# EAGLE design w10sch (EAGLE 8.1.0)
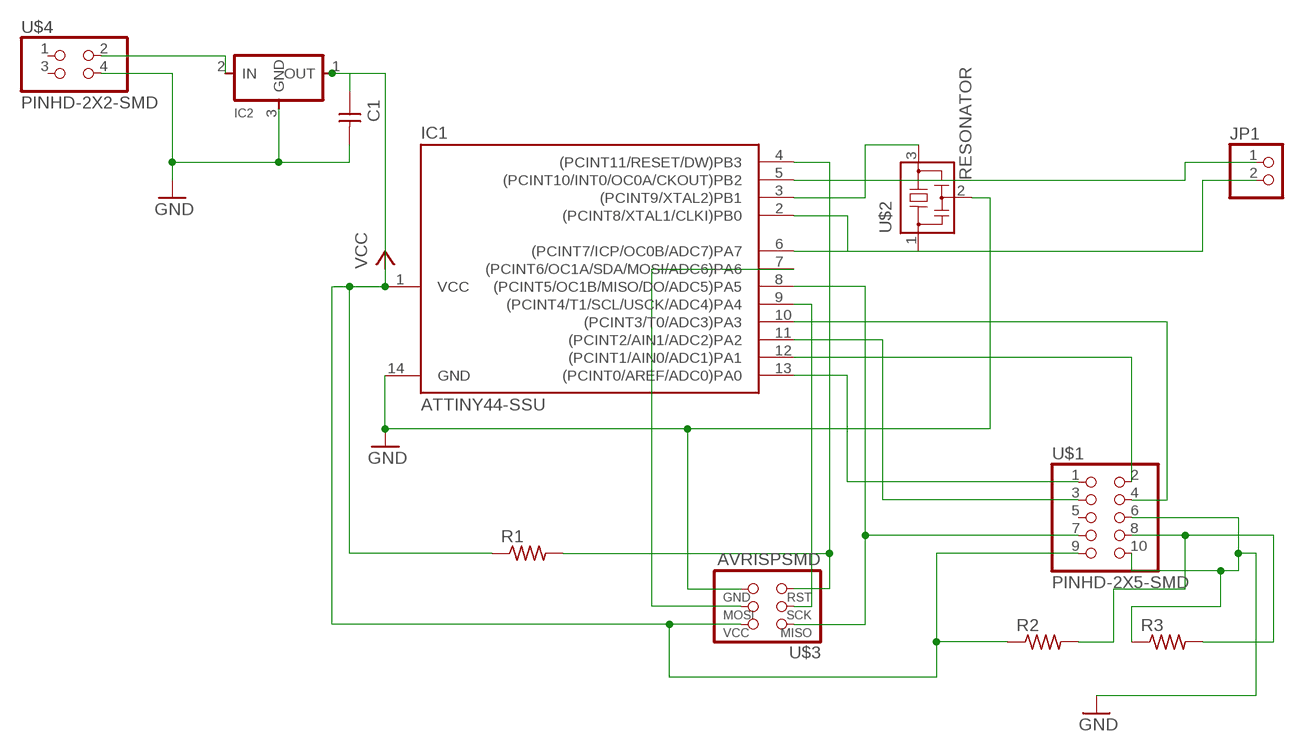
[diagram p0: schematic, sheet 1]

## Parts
C1  CAP-UNPOLARIZEDFAB  [C1206FAB]
IC1  ATTINY44-SSU  [SOIC14]
IC2  REGULATORSOT23  [SOT23]
JP1  PINHD-1X2  [1X02]
R1  RES-US1206FAB  [R1206FAB]
R2  RES-US1206FAB  [R1206FAB]
R3  RES-US1206FAB  [R1206FAB]
U$1  PINHD-2X5-SMD  [2X05SMD]
U$2  RESONATOR  [EFOBM]
U$3  AVRISPSMD  [2X03SMD]
U$4  PINHD-2X2-SMD  [2X02SMD]

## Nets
GND: C1.2 IC1.14(GND) IC2.3(GND) R3.1 U$1.6 U$1.10 U$2.2 U$3.6(GND) U$4.4
N$1: IC1.2((PCINT8/XTAL1/CLKI)PB0) U$2.1
N$2: IC1.3((PCINT9/XTAL2)PB1) U$2.3
N$3: IC2.2(IN) U$4.2
N$4: IC1.7((PCINT6/OC1A/SDA/MOSI/ADC6)PA6) U$3.4(MOSI)
N$5: IC1.9((PCINT4/T1/SCL/USCK/ADC4)PA4) U$3.3(SCK)
N$6: IC1.4((PCINT11/RESET/DW)PB3) R1.2 U$3.5(RST)
N$7: IC1.8((PCINT5/OC1B/MISO/DO/ADC5)PA5) U$1.7 U$3.1(MISO)
N$8: IC1.13((PCINT0/AREF/ADC0)PA0) U$1.1
N$9: IC1.12((PCINT1/AIN0/ADC1)PA1) U$1.2
N$10: IC1.11((PCINT2/AIN1/ADC2)PA2) U$1.3
N$11: IC1.10((PCINT3/T0/ADC3)PA3) U$1.4
N$14: R2.2 R3.2 U$1.8
N$17: IC1.5((PCINT10/INT0/OC0A/CKOUT)PB2) JP1.1
N$18: IC1.6((PCINT7/ICP/OC0B/ADC7)PA7) JP1.2
VCC: C1.1 IC1.1(VCC) IC2.1(OUT) R1.1 R2.1 U$1.9 U$3.2(VCC)
Unconnected: U$1.5 U$4.1 U$4.3

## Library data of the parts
C1 = fab:CAP-UNPOLARIZED
IC1 = fab:ATTINY44
IC2 = fab:REGULATOR
JP1 = pinhead:PINHD-1X2: PIN HEADER
R1-R3 = fab:RES-US: Resistor (US Symbol)
U$1 = fab:PINHD-2X5-SMD
U$2 = fab:RESONATOR
U$3 = fab:AVRISP
U$4 = fab:PINHD-2X2-SMD

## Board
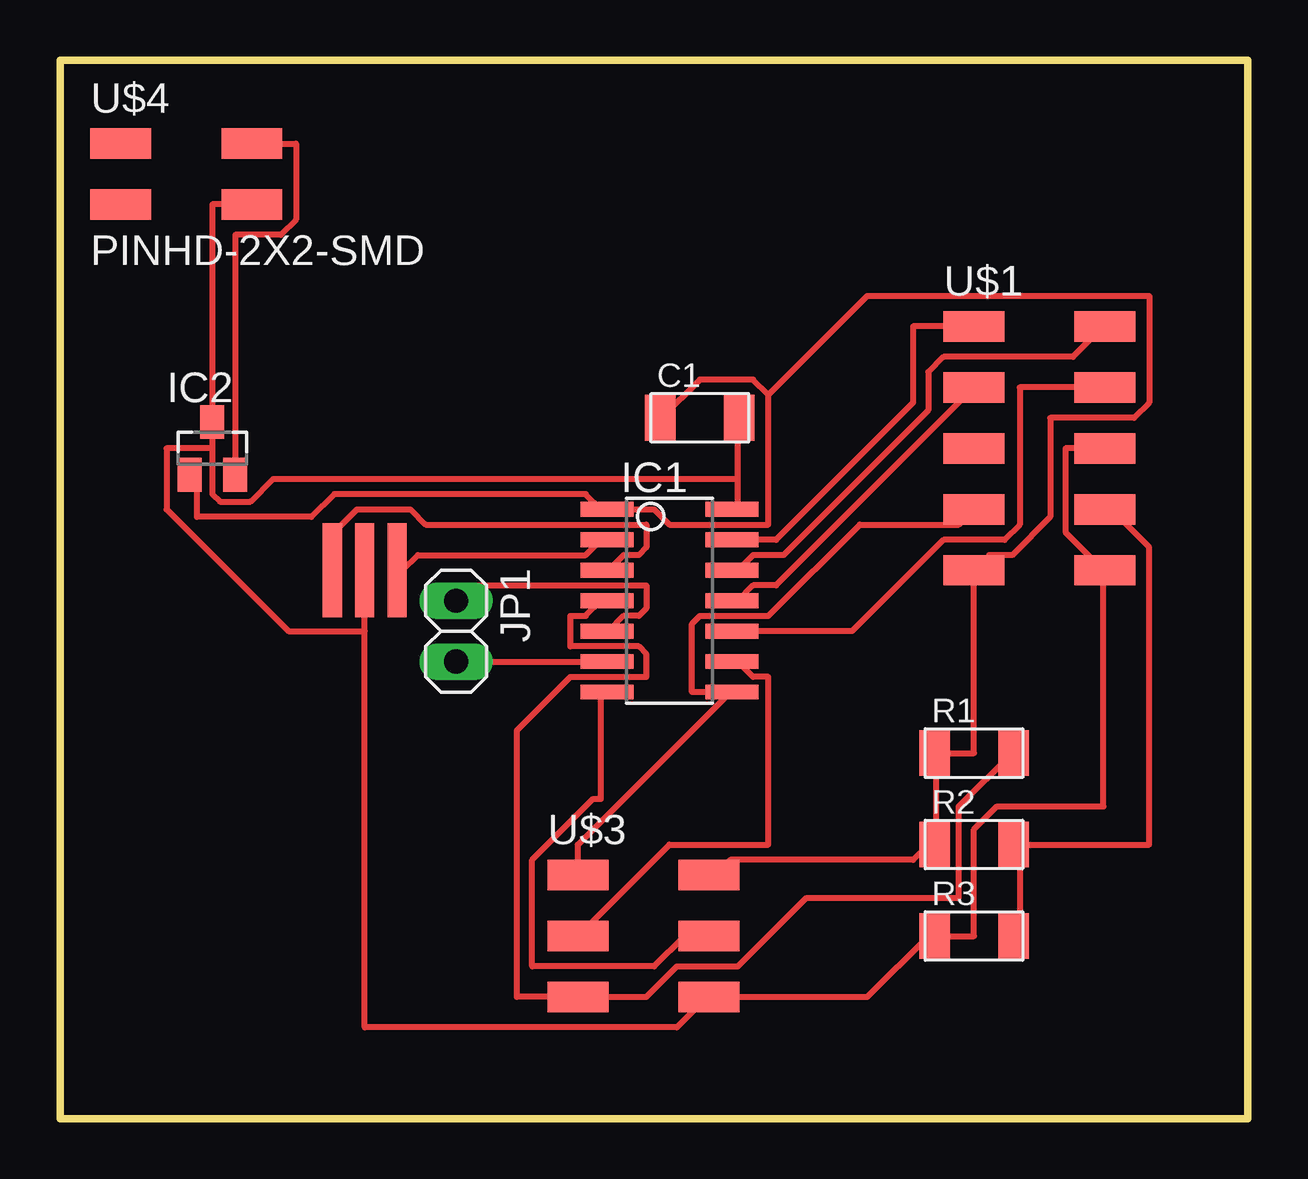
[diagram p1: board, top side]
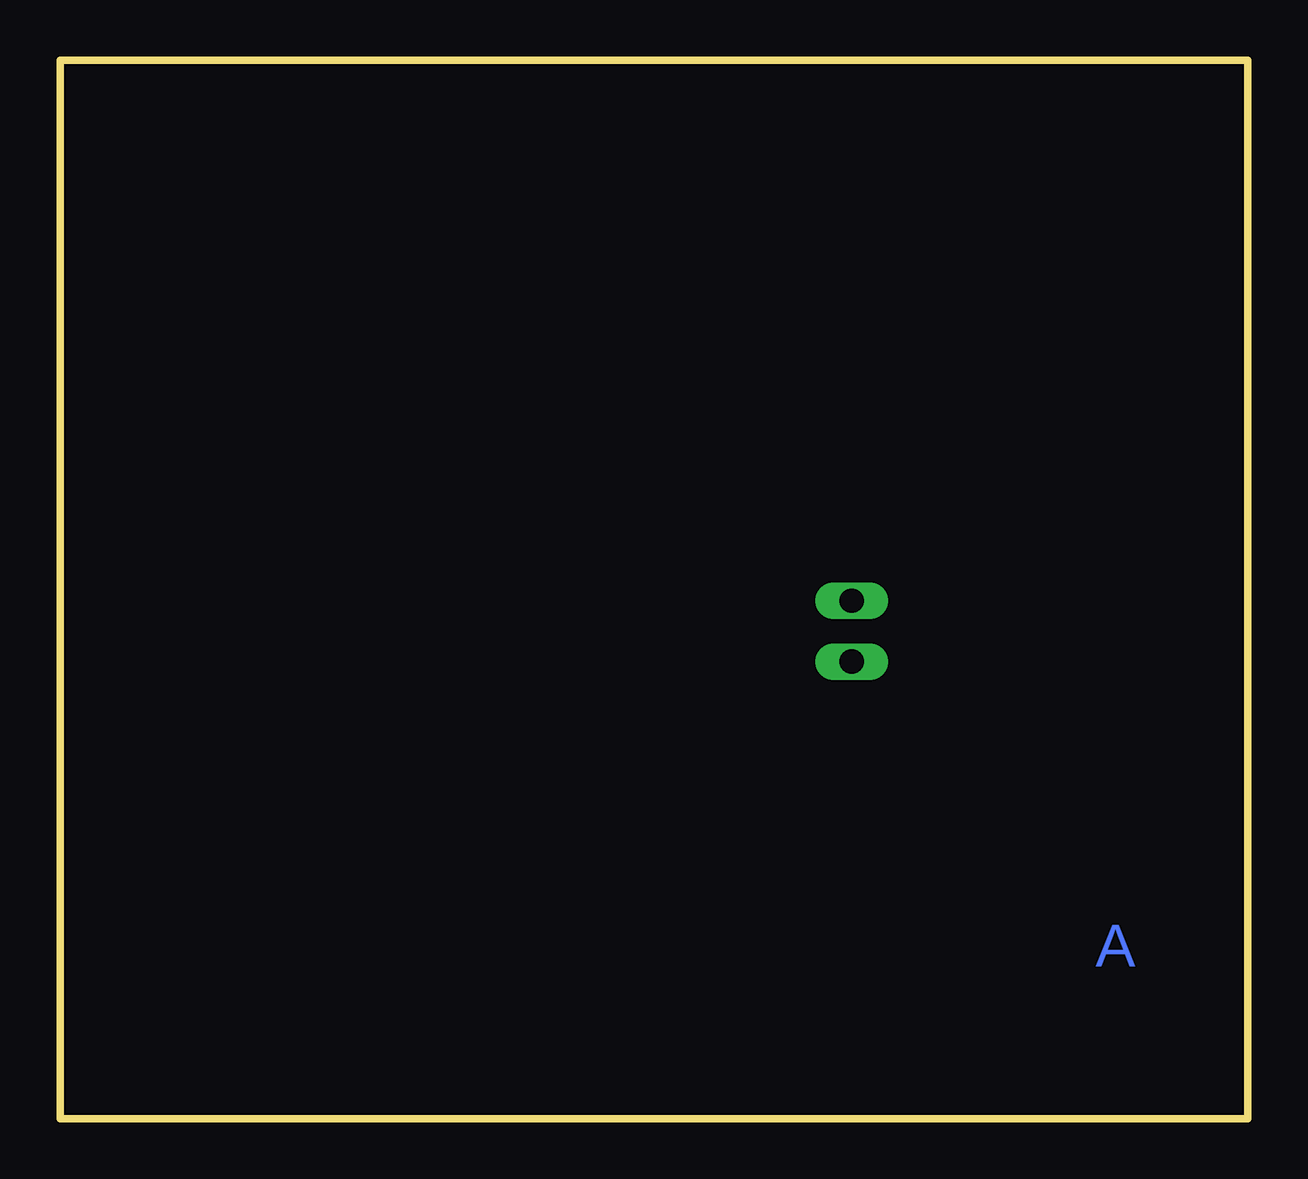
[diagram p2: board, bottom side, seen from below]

Size 49.51 x 44.12 mm. Coordinates in mm from the lower left corner, seen from the top.
Outline: 0,0 49.51,0 49.51,44.12 0,44.12 0,0
Copper layers (1*16): Top 0.035mm / dielectric 1.5mm / Bottom 0.035mm
Design rules "default": minimum track width 10mil, minimum drill 24mil, track to track 8mil, track to pad 8mil, pad to pad 8mil, via to via 8mil, smd to smd 8mil, copper to edge 40mil, drill to drill 8mil, minimum pad ring 10mil, minimum via ring 8mil, stop-mask expansion 4mil, vias tented up to drill 0mil, thermal gap 10mil

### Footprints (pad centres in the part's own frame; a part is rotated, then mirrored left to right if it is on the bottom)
C1206FAB = smd 1.27 x 1.905: 1 -1.651,0; 2 1.651,0
SOIC14 = smd 0.61 x 2.21: 1 -3.81,-2.603; 2 -2.54,-2.603; 3 -1.27,-2.603; 4 0,-2.603; 5 1.27,-2.603; 6 2.54,-2.603; 7 3.81,-2.603; 8 3.81,2.603; 9 2.54,2.603; 10 1.27,2.603; 11 0,2.603; 12 -1.27,2.603; 13 -2.54,2.603; 14 -3.81,2.603
SOT23 = smd 1 x 1.4: 1 -0.95,-1.1; 2 0.95,-1.1; 3 0,1.1
1X02 = drill 1.016 long: 1 -1.27,0; 2 1.27,0
R1206FAB = smd 1.27 x 1.905: 1 -1.651,0; 2 1.651,0
2X05SMD = smd 2.54 x 1.27: 1 -2.54,2.54; 2 2.92,2.54; 3 -2.54,0; 4 2.92,0; 5 -2.54,-2.54; 6 2.92,-2.54; 7 -2.54,-5.08; 8 2.92,-5.08; 9 -2.54,-7.62; 10 2.92,-7.62
EFOBM = smd 0.8 x 3.9: 1 -1.35,0; 2 0,0; 3 1.35,0
2X03SMD = smd 2.54 x 1.27: 1 -2.54,2.54; 2 2.92,2.54; 3 -2.54,0; 4 2.92,0; 5 -2.54,-2.54; 6 2.92,-2.54
2X02SMD = smd 2.54 x 1.27: 1 -2.54,1.27; 2 2.92,1.27; 3 -2.54,-1.27; 4 2.92,-1.27

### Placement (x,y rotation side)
C1  26.67,29.21 0 top
IC1  25.4,21.59 270 top
IC2  6.35,27.94 0 top
JP1  16.51,20.32 270 top
R1  38.1,15.24 0 top
R2  38.1,11.43 0 top
R3  38.1,7.62 0 top
U$1  40.64,30.48 0 top
U$2  12.7,22.86 180 top
U$3  24.13,7.62 0 top
U$4  5.08,39.37 0 top

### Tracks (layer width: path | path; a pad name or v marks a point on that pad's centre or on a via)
GND
  Top 0.254: 28.26,26.67 28.26,25.4 IC1.14 | 28.26,26.67 28.26,29.21 C1.2 | U$4.4 6.35,38.1 IC2.3 6.35,27.94 | 28.26,26.67 8.89,26.67 7.94,25.72 6.67,25.72 6.35,26.04 6.35,27.94 | 12.7,20.32 U$2.2 | 12.7,20.32 9.52,20.32 4.45,25.4 4.45,27.94 6.35,27.94 | 43.5,22.86 41.91,24.45 41.91,27.94 U$1.6 | 43.5,22.86 43.5,13.02 39.05,13.02 38.1,12.06 38.1,7.62 R3.1 36.2,7.62 33.65,5.08 U$3.6 26.99,5.08 25.72,3.81 12.7,3.81 12.7,20.32 | 43.5,22.86 U$1.10
N$1
  Top 0.254: IC1.2 22.54,24.13 21.91,23.49 14.92,23.49 14.29,22.86 U$2.1
N$2
  Top 0.254: IC1.3 22.86,22.86 23.49,23.49 24.13,23.49 24.45,23.81 24.45,24.77 15.24,24.77 14.61,25.4 12.38,25.4 11.43,24.45 11.43,22.86 U$2.3
N$3
  Top 0.254: U$4.2 9.84,40.64 9.84,37.47 9.21,36.83 7.3,36.83 7.3,26.99 IC2.2
N$4
  Top 0.254: U$3.4 26.04,7.62 24.77,6.35 19.69,6.35 19.69,10.8 22.23,13.34 22.54,13.34 22.54,17.78 IC1.7
N$5
  Top 0.254: U$3.3 25.4,11.43 29.53,11.43 29.53,18.41 28.89,18.41 28.26,19.05 IC1.9
N$6
  Top 0.254: R1.2 39.69,15.24 37.46,13.02 37.46,9.21 31.12,9.21 28.26,6.35 25.72,6.35 24.45,5.08 U$3.5 19.05,5.08 19.05,16.19 21.27,18.41 24.45,18.41 24.45,19.37 24.13,19.69 21.27,19.69 21.27,20.95 21.91,20.95 22.54,21.59 IC1.4
N$7
  Top 0.254: 27.94,17.78 21.59,11.43 U$3.1 | U$1.7 37.46,24.77 33.34,24.77 29.53,20.95 26.67,20.95 26.35,20.64 26.35,17.78 27.94,17.78 | 27.94,17.78 IC1.8
N$8
  Top 0.254: IC1.13 29.85,24.13 35.56,29.84 35.56,33.02 U$1.1
N$9
  Top 0.254: IC1.12 28.26,22.86 28.89,23.49 30.16,23.49 36.2,29.53 36.2,31.12 36.83,31.75 42.23,31.75 43.5,33.02 U$1.2
N$10
  Top 0.254: U$1.3 29.85,22.23 28.89,22.23 28.26,21.59 IC1.11
N$11
  Top 0.254: IC1.10 33.02,20.32 36.83,24.13 39.37,24.13 40.01,24.77 40.01,30.48 U$1.4
N$14
  Top 0.254: 40.01,11.43 40.01,7.62 R3.2 | 40.01,11.43 45.4,11.43 45.4,23.81 43.82,25.4 U$1.8 | 40.01,11.43 R2.2
N$17
  Top 0.254: JP1.1 17.15,22.23 24.45,22.23 24.45,21.27 24.13,20.95 23.49,20.95 22.86,20.32 IC1.5
N$18
  Top 0.254: JP1.2 IC1.6
VCC
  Top 0.254: 36.51,15.24 36.51,11.43 R2.1 36.2,11.43 35.56,10.8 27.94,10.8 27.3,10.16 U$3.2 | 36.51,15.24 38.1,15.24 U$1.9 38.74,23.49 39.69,23.49 41.27,25.08 41.27,29.21 44.77,29.21 45.4,29.84 45.4,34.29 33.65,34.29 29.53,30.16 | 36.51,15.24 R1.1 | IC2.1 5.72,26.67 5.72,25.08 10.48,25.08 11.43,26.04 21.91,26.04 22.54,25.4 IC1.1 24.77,25.4 25.4,24.77 29.53,24.77 29.53,30.16 | 29.53,30.16 28.89,30.8 26.67,30.8 25.08,29.21 C1.1

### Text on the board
Bottom: A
